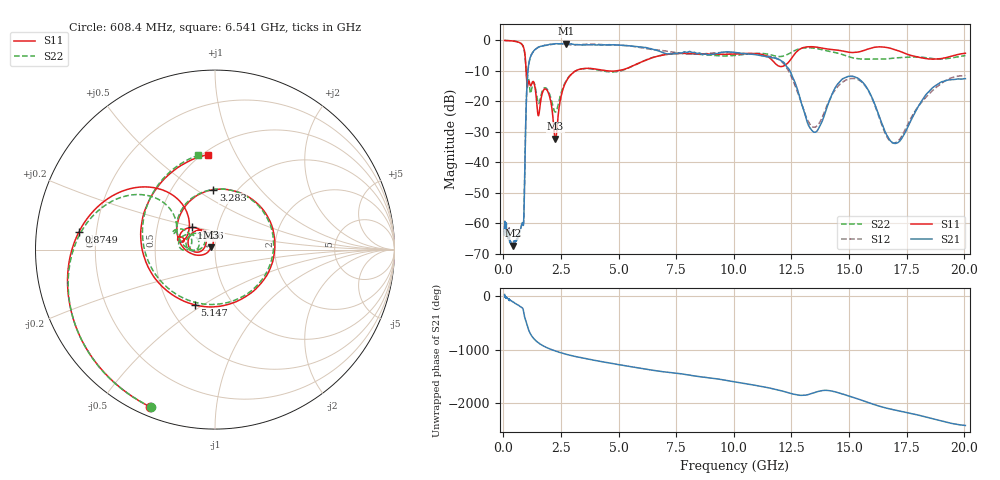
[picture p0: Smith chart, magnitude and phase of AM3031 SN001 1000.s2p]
# Hz S DB R 50
!freq MagS11 AngS11 MagS21 AngS21 MagS12 AngS12 MagS22 AngS22
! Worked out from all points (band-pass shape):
!   1601 points, 50 MHz to 20.05 GHz, reference 50 ohm
!   highest |S21| = -1.05 dB at 2.702 GHz (marker M1); lowest = -67.4 dB at 421.4 MHz (marker M2)
!   |S21| within 3 dB of the highest: 1.264 GHz to 6.922 GHz (5.657 GHz wide, 138 % of centre); 9.401 GHz to 10.13 GHz (730 MHz wide, 7.47 % of centre)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
!   lowest |S11| = -32.2 dB at 2.257 GHz (marker M3), VSWR 1.05, Z = 47.9 + j1.2 ohm
!   |S11| at or under -10 dB: 982.1 MHz to 3.133 GHz (2.151 GHz wide, 105 % of centre); 4.506 GHz to 4.898 GHz (392.2 MHz wide, 8.34 % of centre)
!   |S22| runs from -23.6 to 0.0 dB; largest |S21 - S12| = 0.067
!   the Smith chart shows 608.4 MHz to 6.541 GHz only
!   S11 on the Smith chart (normalised r, x): 608.4 MHz: 0.04, -0.67; 874.9 MHz: 0.13, +0.06; 1.356 GHz: 0.75, +0.19; 3.283 GHz: 0.79, +0.59; 5.147 GHz: 0.67, -0.46; 6.541 GHz: 0.53, +0.78
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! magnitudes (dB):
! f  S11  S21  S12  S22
! 50 MHz  0.0  -61.8  -61.5  0.0
! 135.9 MHz  -0.1  -62.7  -63.0  0.0
! 369.6 MHz  -0.1  -67.0  -67.0  -0.2
! 421.4 MHz  -0.2  -67.4  -66.6  -0.2
! 608.4 MHz  -0.5  -65.2  -65.4  -0.5
! 874.9 MHz  -2.3  -59.8  -59.7  -2.4
! 1.005 GHz  -13.4  -17.3  -17.2  -12.0
! 1.356 GHz  -14.9  -3.1  -3.2  -14.5
! 1.518 GHz  -24.8  -2.2  -2.2  -20.7
! 1.929 GHz  -16.9  -1.5  -1.5  -16.4
! 2.257 GHz  -32.2  -1.1  -1.2  -23.6
! 2.702 GHz  -13.8  -1.0  -1.3  -13.5
! 2.722 GHz  -13.5  -1.1  -1.3  -13.2
! 3.283 GHz  -9.5  -1.4  -1.4  -9.6
! 5.147 GHz  -9.7  -1.6  -1.6  -9.9
! 6.541 GHz  -5.5  -3.0  -3.0  -5.5
! 7.402 GHz  -4.3  -4.3  -4.0  -4.3
! 11.87 GHz  -8.0  -6.1  -5.9  -5.2
! 13.48 GHz  -2.1  -30.1  -28.5  -2.5
! 15.2 GHz  -4.0  -11.9  -12.5  -5.8
! 16.94 GHz  -2.9  -33.8  -33.7  -5.8
! 20.05 GHz  -4.2  -12.6  -11.5  -5.0
